PROGRAM P_Prog7
VAR

	fbKL6401 		: FB_LON_KL6401;

	fbREAD_191		: FB_READ_191_SNVT_log_status;
	fbSEND_191		: FB_SEND_191_SNVT_log_status;

	fbREAD_192		: FB_READ_192_SNVT_time_stamp_p;
	fbSEND_192		: FB_SEND_192_SNVT_time_stamp_p;

	fbREAD_193		: FB_READ_193_SNVT_log_fx_request;
	fbSEND_193		: FB_SEND_193_SNVT_log_fx_request;

	fbREAD_194		: FB_READ_194_SNVT_log_fx_status;
	fbSEND_194		: FB_SEND_194_SNVT_log_fx_status;

	fbREAD_195		: FB_READ_195_SNVT_log_request;
	fbSEND_195		: FB_SEND_195_SNVT_log_request;

	fbREAD_196		: FB_READ_196_SNVT_enthalpy_d;
	fbSEND_196		: FB_SEND_196_SNVT_enthalpy_d;

	fbREAD_197		: FB_READ_197_SNVT_amp_ac_mil;
	fbSEND_197		: FB_SEND_197_SNVT_amp_ac_mil;

	fbREAD_198		: FB_READ_198_SNVT_time_hour_p;
	fbSEND_198		: FB_SEND_198_SNVT_time_hour_p;

	fbREAD_199		: FB_READ_199_SNVT_lamp_status;
	fbSEND_199		: FB_SEND_199_SNVT_lamp_status;

	fbREAD_200		: FB_READ_200_SNVT_environment;
	fbSEND_200		: FB_SEND_200_SNVT_environment;

	fbREAD_201		: FB_READ_201_SNVT_geo_loc;
	fbSEND_201		: FB_SEND_201_SNVT_geo_loc;
END_VAR

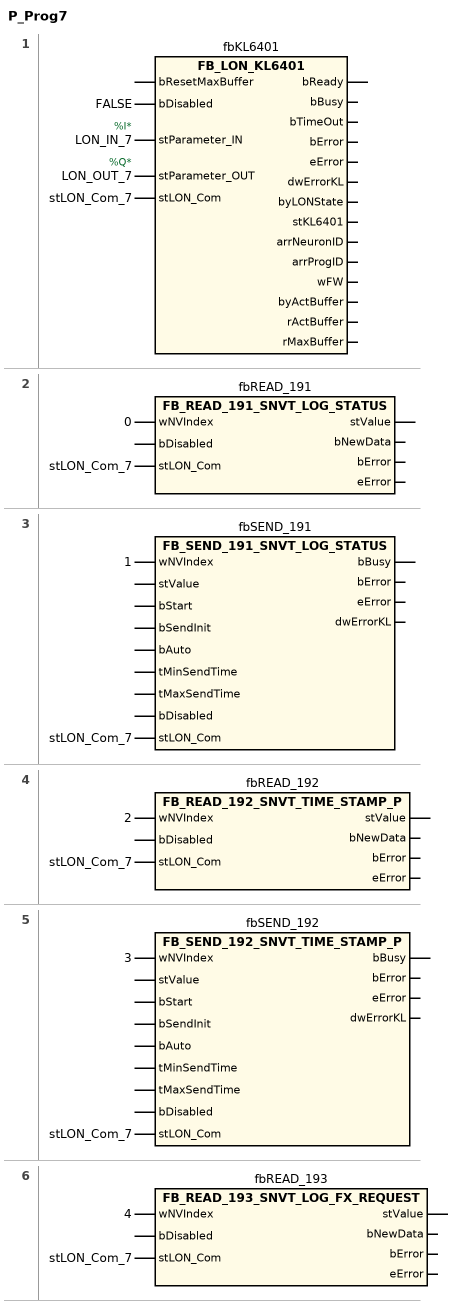
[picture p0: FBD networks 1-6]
// NETWORK 1
//   LON_IN_7: AT %I*
//   LON_OUT_7: AT %Q*
fbKL6401(
    bDisabled := FALSE,
    stParameter_IN := LON_IN_7,
    stParameter_OUT := LON_OUT_7,
    stLON_Com := stLON_Com_7); // FB_LON_KL6401

// NETWORK 2
fbREAD_191(wNVIndex := 0, stLON_Com := stLON_Com_7); // FB_READ_191_SNVT_LOG_STATUS

// NETWORK 3
fbSEND_191(wNVIndex := 1, stLON_Com := stLON_Com_7); // FB_SEND_191_SNVT_LOG_STATUS

// NETWORK 4
fbREAD_192(wNVIndex := 2, stLON_Com := stLON_Com_7); // FB_READ_192_SNVT_TIME_STAMP_P

// NETWORK 5
fbSEND_192(wNVIndex := 3, stLON_Com := stLON_Com_7); // FB_SEND_192_SNVT_TIME_STAMP_P

// NETWORK 6
fbREAD_193(wNVIndex := 4, stLON_Com := stLON_Com_7); // FB_READ_193_SNVT_LOG_FX_REQUEST

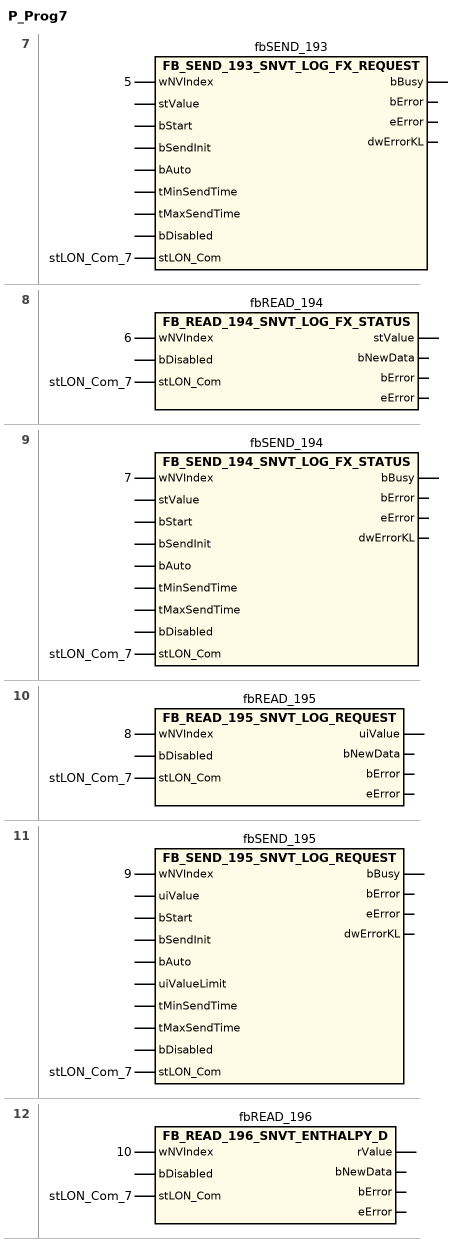
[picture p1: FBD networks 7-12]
// NETWORK 7
fbSEND_193(wNVIndex := 5, stLON_Com := stLON_Com_7); // FB_SEND_193_SNVT_LOG_FX_REQUEST

// NETWORK 8
fbREAD_194(wNVIndex := 6, stLON_Com := stLON_Com_7); // FB_READ_194_SNVT_LOG_FX_STATUS

// NETWORK 9
fbSEND_194(wNVIndex := 7, stLON_Com := stLON_Com_7); // FB_SEND_194_SNVT_LOG_FX_STATUS

// NETWORK 10
fbREAD_195(wNVIndex := 8, stLON_Com := stLON_Com_7); // FB_READ_195_SNVT_LOG_REQUEST

// NETWORK 11
fbSEND_195(wNVIndex := 9, stLON_Com := stLON_Com_7); // FB_SEND_195_SNVT_LOG_REQUEST

// NETWORK 12
fbREAD_196(wNVIndex := 10, stLON_Com := stLON_Com_7); // FB_READ_196_SNVT_ENTHALPY_D

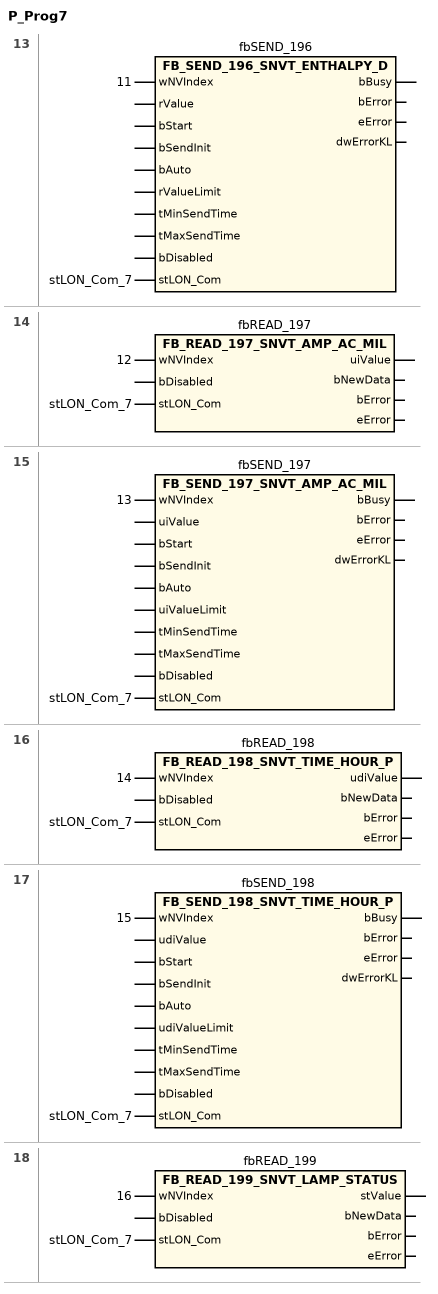
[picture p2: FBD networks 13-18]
// NETWORK 13
fbSEND_196(wNVIndex := 11, stLON_Com := stLON_Com_7); // FB_SEND_196_SNVT_ENTHALPY_D

// NETWORK 14
fbREAD_197(wNVIndex := 12, stLON_Com := stLON_Com_7); // FB_READ_197_SNVT_AMP_AC_MIL

// NETWORK 15
fbSEND_197(wNVIndex := 13, stLON_Com := stLON_Com_7); // FB_SEND_197_SNVT_AMP_AC_MIL

// NETWORK 16
fbREAD_198(wNVIndex := 14, stLON_Com := stLON_Com_7); // FB_READ_198_SNVT_TIME_HOUR_P

// NETWORK 17
fbSEND_198(wNVIndex := 15, stLON_Com := stLON_Com_7); // FB_SEND_198_SNVT_TIME_HOUR_P

// NETWORK 18
fbREAD_199(wNVIndex := 16, stLON_Com := stLON_Com_7); // FB_READ_199_SNVT_LAMP_STATUS

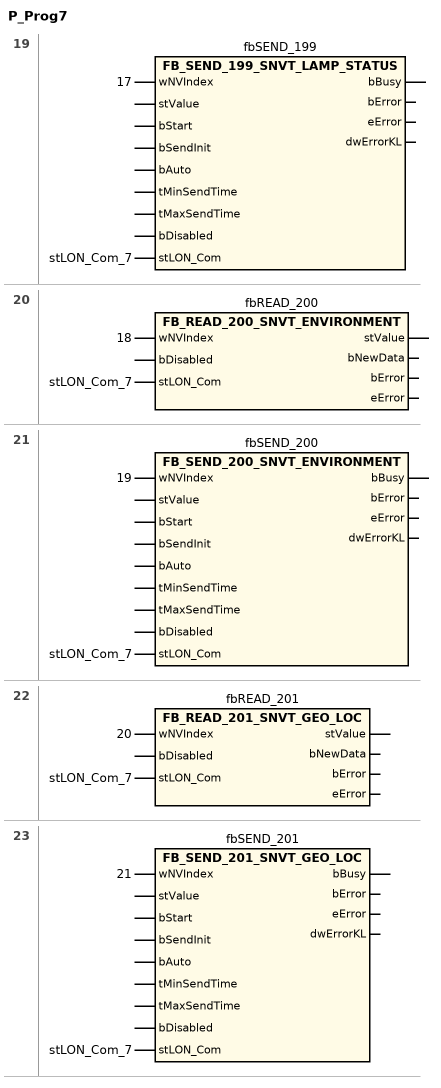
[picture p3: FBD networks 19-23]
// NETWORK 19
fbSEND_199(wNVIndex := 17, stLON_Com := stLON_Com_7); // FB_SEND_199_SNVT_LAMP_STATUS

// NETWORK 20
fbREAD_200(wNVIndex := 18, stLON_Com := stLON_Com_7); // FB_READ_200_SNVT_ENVIRONMENT

// NETWORK 21
fbSEND_200(wNVIndex := 19, stLON_Com := stLON_Com_7); // FB_SEND_200_SNVT_ENVIRONMENT

// NETWORK 22
fbREAD_201(wNVIndex := 20, stLON_Com := stLON_Com_7); // FB_READ_201_SNVT_GEO_LOC

// NETWORK 23
fbSEND_201(wNVIndex := 21, stLON_Com := stLON_Com_7); // FB_SEND_201_SNVT_GEO_LOC

END_PROGRAM
